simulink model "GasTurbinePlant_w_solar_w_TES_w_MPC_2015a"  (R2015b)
settings: Solver=ode45  StartTime=0.0  StopTime=120  FixedStep=0.05  MinStep=0.000001  RelTol=1e-3
InitFcn:
  | main()
StopFcn:
  | Plot_Step_Test()
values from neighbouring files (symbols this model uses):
  A0 = .945    (= 0.945)    [main.m]
  A1 = -7.8    [main.m]
  A2 = 39    [main.m]
  A_air = (1 - pct) * A_tank    (= 5.890486125)    [main.m]
  A_lm = (A_outer - A_inner) / log(A_outer / A_inner)    [main.m]
  Ac = pct * A_tank    (= 13.744467625)    [main.m]
  B = [-0.22824; 3.3801e5; -3.4738e7; 110.88; -2378.1]    [main.m]
  C = [2.8958e04; 9.3900e03; 3.0120e03; 7.5800e03; 1.4840e03]    [main.m]
  Cp_air = ones(n_tes,1)*300    [main.m]
  Cp_stone = ones(n_tes,1)*1584    [main.m]
  Cpc = 1.005    [main.m]
  Cph = 1.157    [main.m]
  d_rec = 5    [main.m]
  dHst = Hsh - Hcond    (= 811.3)    [main.m]
  dHtot = (Hsh-Hsv)+Hfg+Cpw*delTbfw    (= 2789.54)    [main.m]
  dp = 0.15    [main.m]
  emiss_rec = 0.1    [main.m]
  epsilon = 0.96    [main.m]
  eta_c = 0.86    [main.m]
  eta_comb = 0.99    [main.m]
  eta_HRSG = 0.95    [main.m]
  eta_st = 0.95    [main.m]
  eta_t = 0.89    [main.m]
  F = [1.4250E-06; 5.0390E-01; 1.0830E+02; 0]    [main.m]
  gamma_c = 1.4    [main.m]
  gamma_h = 1.33    [main.m]
  h = ones(n_tes,1)    [main.m]    (also in apm_linprog.m = [hi,hj,hv]'; apm_quadprog.m = [hi,hj,hv]')
  h_node_rec = 2    [main.m]
  k_air = ones(n_tes,1)    [main.m]
  k_stone = 1.7    [main.m]
  LHV = 46000    [main.m]
  m_air = zeros(n_tes,1)    [main.m]
  m_stone = ones(n_tes,1) * V_tank * rho_stone * pct / n_tes    [main.m]
  mu_air2 = zeros(n_tes,1)    [main.m]
  MW_air = 28.97    [main.m]
  n_rec = 10    [main.m]
  n_tes = 10    [main.m]
  Nu = ones(n_tes,1)    [main.m]
  Pa = 101.325    [main.m]
  Pa0 = 101.325    [main.m]
  pct = 0.7    [main.m]
  PR = 15.4    [main.m]
  Pr = ones(n_tes,1)    [main.m]
  q_cond = zeros(n_tes,1)    [main.m]
  q_conv = zeros(n_tes,1)    [main.m]
  q_external = zeros(n_tes,1)    [main.m]
  q_rad = zeros(n_tes,1)    [main.m]
  R = 8.314    [main.m]
  R2 = 0.08206    [main.m]
  Re = ones(n_tes,1)    [main.m]
  rho_air = zeros(n_tes,1)    [main.m]
  SA = 137.445    [main.m]
  sig = 5.6704e-11    [main.m]
  sigma = 5.67e-8    (= 5.67e-08)    [main.m]
  T_air0 = ones(n_tes,1)*298    [main.m]
  T_ref = 298    [main.m]
  T_stone0 = ones(n_tes,1)*298    [main.m]
  T_wall_outer = ones(n_tes,1)*298    [main.m]
  Ta0 = 298.15    [main.m]
  Tao = 298    [main.m]
  theta0 = 11.6    [main.m]
  thetaMAX = 85    [main.m]
  Trec0 = ones(n_rec,1)*550    [main.m]
  U = .010    (= 0.01)    [main.m]
  U_wall = 0.1    [main.m]
  v_air = ones(n_tes,1)    [main.m]
  V_tank = A_tank * len    (= 196.3495375)    [main.m]
  Vol_air = ones(n_tes,1)    [main.m]
  w_rec = 10    [main.m]
  Wfn = 10.2    [main.m]
  Wn = 537    [main.m]
  x = len / n_tes    (= 1)    [main.m]
libraries: simulink x3

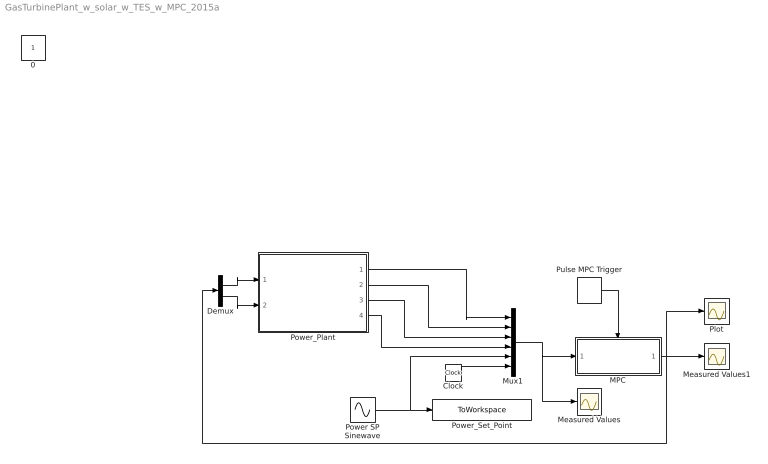
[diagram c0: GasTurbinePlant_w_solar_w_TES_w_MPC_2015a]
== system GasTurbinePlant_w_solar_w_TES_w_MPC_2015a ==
  Clock : Clock
  Demux : Demux  Outputs=2
  MPC : Subsystem  TreatAsAtomicUnit=on
  Measured Values : Scope
  Measured Values1 : Scope
  Mux1 : Mux  Inputs=6
  Plot : Scope
  Power SP Sinewave : Sin  Amplitude=10  Bias=90  Frequency=1/250*20  SampleTime=0
  Power_Plant : Subsystem
  Power_Set_Point : ToWorkspace  VariableName=Power_Set_Point  SaveFormat=Timeseries  SampleTime=-1
  Pulse MPC Trigger : DiscretePulseGenerator  PulseType=Time based  Period=5  PulseWidth=25
  0 : Constant  IOType=siggen
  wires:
  Mux1/1 -> Measured Values/1, MPC/1(In1)
  Pulse MPC Trigger/1 -> MPC/Trigger
  MPC/1(Out1) -> Measured Values1/1, Plot/1, Demux/1
  Demux/1 -> Power_Plant/1(IGV_Input)
  Demux/2 -> Power_Plant/2(Fuel_Input)
  Power_Plant/1(Power_Total) -> Mux1/1
  Power_Plant/3("Te ") -> Mux1/3
  Power_Plant/4("W ") -> Mux1/4
  Clock/1 -> Mux1/6
  Power SP Sinewave/1 -> Power_Set_Point/1, Mux1/5
  Power_Plant/2("Tf ") -> Mux1/2

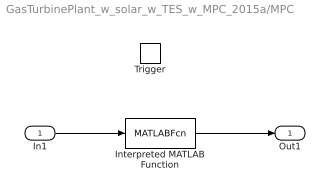
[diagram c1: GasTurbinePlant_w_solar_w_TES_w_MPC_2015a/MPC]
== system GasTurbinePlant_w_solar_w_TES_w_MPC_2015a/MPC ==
  In1 : Inport
  Trigger : TriggerPort
  Interpreted MATLAB Function : MATLABFcn  MATLABFcn=mpc  OutputDimensions=2
  Out1 : Outport  InitialOutput=[50 5]
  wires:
  In1/1 -> Interpreted MATLAB Function/1
  Interpreted MATLAB Function/1 -> Out1/1

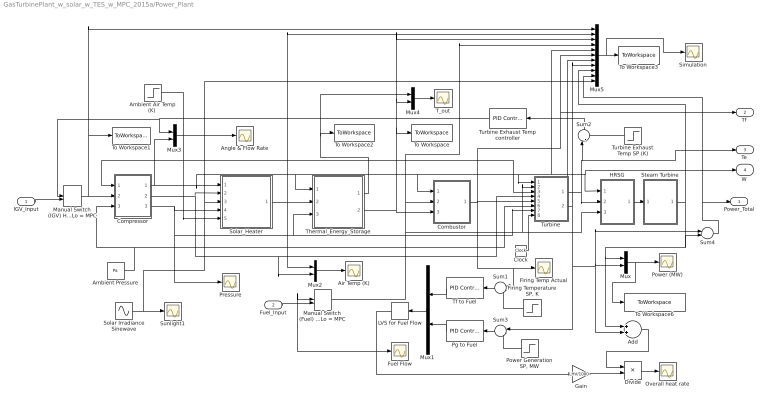
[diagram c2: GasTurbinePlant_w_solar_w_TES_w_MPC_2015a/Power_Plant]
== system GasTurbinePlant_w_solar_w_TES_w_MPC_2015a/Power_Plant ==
  IGV_Input : Inport
  Fuel_Input : Inport  Port=2
  Add : Sum
  Air Temp (K) : Scope
  "Ambient Air Temp (K) " : Step  Time=0  Before=298  After=298  SampleTime=0
  Ambient Pressure : Constant  Value=Pa
  Angle & Flow Rate : Scope
  Clock : Clock
  Combustor : Subsystem
  Compressor : Subsystem
  Divide : Product  Inputs=*/
  Firing Temp Actual : Scope
  "Firing Temperature SP, K" : Step  Time=10  Before=1370  After=1370  SampleTime=0
  Fuel Flow : Scope
  Gain : Gain  Gain=LHV/1000
  HRSG : Subsystem
  LVS for Fuel Flow : MinMax
  Manual Switch (Fuel) Hi = PID Lo = MPC : ManualSwitch  CurrentSetting=0
  Manual Switch (IGV) Hi = PID Lo = MPC : ManualSwitch  CurrentSetting=0
  Mux{,1..4} (5 alike) : Mux  Inputs=2
  Mux5 : Mux  Inputs=11
  Overall heat rate : Scope
  Pg to Fuel : simulink/Continuous/PID Controller  Controller=PID  TimeDomain=Discrete-time  SampleTime=1/60*6  IntegratorMethod=Forward Euler  FilterMethod=Forward Euler  Form=Ideal  UseFilter=on  ControllerParametersSource=internal  P=1/15  I=1  D=0  N=1  InitialConditionSource=internal  InitialConditionForIntegrator=50  InitialConditionForFilter=0  ExternalReset=none  LimitOutput=on  UpperSaturationLimit=12  LowerSaturationLimit=0.5  LinearizeAsGain=off  AntiWindupMode=clamping  Kb=1  TrackingMode=off  Kt=1  PParamMin=[]  PParamMax=[]  IParamMin=[]  IParamMax=[]  DParamMin=[]  DParamMax=[]  NParamMin=[]  NParamMax=[]  KbParamMin=[]  KbParamMax=[]  KtParamMin=[]  KtParamMax=[]  POutMin=[]  POutMax=[]  IOutMin=[]  IOutMax=[]  DOutMin=[]  DOutMax=[]  NOutMin=[]  NOutMax=[]  KbOutMin=[]  KbOutMax=[]  KtOutMin=[]  KtOutMax=[]  IntegratorOutMin=[]  IntegratorOutMax=[]  FilterOutMin=[]  FilterOutMax=[]  SumOutMin=[]  SumOutMax=[]  SumI1OutMin=[]  SumI1OutMax=[]  SumI2OutMin=[]  SumI2OutMax=[]  SumI3OutMin=[]  SumI3OutMax=[]  SumDOutMin=[]  SumDOutMax=[]  SaturationOutMin=[]  SaturationOutMax=[]  IntegratorContinuousStateAttributes=''  IntegratorStateMustResolveToSignalObject=off  IntegratorRTWStateStorageClass=Auto  FilterContinuousStateAttributes=''  FilterStateMustResolveToSignalObject=off  FilterRTWStateStorageClass=Auto  DifferentiatorICPrevScaledInput=0  DifferentiatorOutMin=[]  DifferentiatorOutMax=[]
  Power (MW) : Scope
  "Power Generation SP, MW" : Step  Time=40  Before=230  After=230  SampleTime=0
  Pressure : Scope
  Simulation : Scope
  Solar Irradiance Sinewave : Sin  Amplitude=500  Bias=500  Frequency=1/250*20  SampleTime=0
  Solar_Heater : Subsystem
  Steam Turbine : Subsystem
  Sum1 : Sum  Inputs=|-+
  Sum2 : Sum  Inputs=|-+
  Sum3 : Sum  Inputs=|-+
  Sum4 : Sum  Inputs=|++
  Sunlight1 : Scope
  T_out : Scope
  Tf to Fuel : simulink/Continuous/PID Controller  Controller=PID  TimeDomain=Discrete-time  SampleTime=1/60*6  IntegratorMethod=Forward Euler  FilterMethod=Forward Euler  Form=Ideal  UseFilter=on  ControllerParametersSource=internal  P=1/20  I=1  D=0  N=1  InitialConditionSource=internal  InitialConditionForIntegrator=200  InitialConditionForFilter=0  ExternalReset=none  LimitOutput=on  UpperSaturationLimit=12  LowerSaturationLimit=0.5  LinearizeAsGain=off  AntiWindupMode=clamping  Kb=1  TrackingMode=off  Kt=1  PParamMin=[]  PParamMax=[]  IParamMin=[]  IParamMax=[]  DParamMin=[]  DParamMax=[]  NParamMin=[]  NParamMax=[]  KbParamMin=[]  KbParamMax=[]  KtParamMin=[]  KtParamMax=[]  POutMin=[]  POutMax=[]  IOutMin=[]  IOutMax=[]  DOutMin=[]  DOutMax=[]  NOutMin=[]  NOutMax=[]  KbOutMin=[]  KbOutMax=[]  KtOutMin=[]  KtOutMax=[]  IntegratorOutMin=[]  IntegratorOutMax=[]  FilterOutMin=[]  FilterOutMax=[]  SumOutMin=[]  SumOutMax=[]  SumI1OutMin=[]  SumI1OutMax=[]  SumI2OutMin=[]  SumI2OutMax=[]  SumI3OutMin=[]  SumI3OutMax=[]  SumDOutMin=[]  SumDOutMax=[]  SaturationOutMin=[]  SaturationOutMax=[]  IntegratorContinuousStateAttributes=''  IntegratorStateMustResolveToSignalObject=off  IntegratorRTWStateStorageClass=Auto  FilterContinuousStateAttributes=''  FilterStateMustResolveToSignalObject=off  FilterRTWStateStorageClass=Auto  DifferentiatorICPrevScaledInput=0  DifferentiatorOutMin=[]  DifferentiatorOutMax=[]
  Thermal_Energy_Storage : Subsystem
  To Workspace : ToWorkspace  VariableName=T_stone_out  SaveFormat=Timeseries  SampleTime=-1
  To Workspace1 : ToWorkspace  VariableName=IGV_Angle  SaveFormat=Timeseries  SampleTime=-1
  To Workspace2 : ToWorkspace  VariableName=T_air_out  SaveFormat=Timeseries  SampleTime=-1
  To Workspace3 : ToWorkspace  VariableName=Plant_Data  SaveFormat=Timeseries  SampleTime=-1
  To Workspace6 : ToWorkspace  VariableName=Power  SaveFormat=Timeseries  SampleTime=-1
  Turbine : Subsystem
  Turbine Exhaust Temp SP (K) : Step  Time=40  Before=750  After=750  SampleTime=0
  Turbine Exhaust Temp controller : simulink/Continuous/PID Controller  Controller=PID  TimeDomain=Discrete-time  SampleTime=1/60*6  IntegratorMethod=Forward Euler  FilterMethod=Forward Euler  Form=Parallel  UseFilter=on  ControllerParametersSource=internal  P=-1.5  I=-1  D=0  N=1  InitialConditionSource=internal  InitialConditionForIntegrator=75  InitialConditionForFilter=0  ExternalReset=none  LimitOutput=on  UpperSaturationLimit=88  LowerSaturationLimit=57  LinearizeAsGain=off  AntiWindupMode=clamping  Kb=1  TrackingMode=off  Kt=1  PParamMin=[]  PParamMax=[]  IParamMin=[]  IParamMax=[]  DParamMin=[]  DParamMax=[]  NParamMin=[]  NParamMax=[]  KbParamMin=[]  KbParamMax=[]  KtParamMin=[]  KtParamMax=[]  POutMin=[]  POutMax=[]  IOutMin=[]  IOutMax=[]  DOutMin=[]  DOutMax=[]  NOutMin=[]  NOutMax=[]  KbOutMin=[]  KbOutMax=[]  KtOutMin=[]  KtOutMax=[]  IntegratorOutMin=[]  IntegratorOutMax=[]  FilterOutMin=[]  FilterOutMax=[]  SumOutMin=[]  SumOutMax=[]  SumI1OutMin=[]  SumI1OutMax=[]  SumI2OutMin=[]  SumI2OutMax=[]  SumI3OutMin=[]  SumI3OutMax=[]  SumDOutMin=[]  SumDOutMax=[]  SaturationOutMin=[]  SaturationOutMax=[]  IntegratorContinuousStateAttributes=''  IntegratorStateMustResolveToSignalObject=off  IntegratorRTWStateStorageClass=Auto  FilterContinuousStateAttributes=''  FilterStateMustResolveToSignalObject=off  FilterRTWStateStorageClass=Auto  DifferentiatorICPrevScaledInput=0  DifferentiatorOutMin=[]  DifferentiatorOutMax=[]
  Power_Total : Outport
  "Tf " : Outport  Port=2
  "Te " : Outport  Port=3
  "W " : Outport  Port=4
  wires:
  HRSG/1(msteam) -> Steam Turbine/1(msteam)
  Ambient Pressure/1 -> Turbine/6(Pa), Compressor/3(Pa)
  Combustor/1(Tf) -> Sum1/1, Firing Temp Actual/1, Turbine/5(Tf), Mux5/6, "Tf "/1
  Turbine/1(Te) -> HRSG/2(Te), "Te "/1, Sum2/1, Mux5/7
  "Ambient Air Temp (K) "/1 -> Compressor/1(Ta), Turbine/3(Ti), Solar_Heater/5(Ta)
  Turbine Exhaust Temp controller/1 -> Manual Switch (IGV) Hi = PID Lo = MPC/1, Mux3/1
  Steam Turbine/1(Pst) -> Mux5/9, Sum4/2, Mux/1, Add/1
  Mux/1 -> To Workspace6/1, Power (MW)/1
  Sum2/1 -> Turbine Exhaust Temp controller/1
  Turbine Exhaust Temp SP (K)/1 -> Sum2/2
  Sum1/1 -> Tf to Fuel/1
  "Firing Temperature SP, K"/1 -> Sum1/2
  Turbine/2(Pg) -> Sum3/1, Sum4/1, Mux/2, Add/2, Mux5/8
  Sum3/1 -> Pg to Fuel/1
  "Power Generation SP, MW"/1 -> Sum3/2
  Mux1/1 -> LVS for Fuel Flow/1
  Tf to Fuel/1 -> Mux1/1
  Pg to Fuel/1 -> Mux1/2
  LVS for Fuel Flow/1 -> Manual Switch (Fuel) Hi = PID Lo = MPC/1, Gain/1, Fuel Flow/1
  Add/1 -> Divide/1
  Gain/1 -> Divide/2
  Divide/1 -> Overall heat rate/1
  Compressor/2(Td) -> Mux2/2, Turbine/4(Td), Solar_Heater/2(Td)
  Compressor/1(W) -> Mux3/2, Solar_Heater/1(W), HRSG/1(W), "W "/1, Mux5/5, Turbine/1(W), Combustor/1(W), Thermal_Energy_Storage/1(W)
  Compressor/3(Pd) -> Solar_Heater/4(P), Turbine/7(Pd), Thermal_Energy_Storage/3(P), Pressure/1
  Solar_Heater/1(Tair_out) -> Mux5/2, Mux2/1, Thermal_Energy_Storage/2(T_air_in)
  Mux2/1 -> Air Temp (K)/1
  Thermal_Energy_Storage/2(T_air_out) -> Mux4/2, Mux5/3, To Workspace/1, Combustor/3(Td)
  Thermal_Energy_Storage/1(T_stone_out) -> To Workspace2/1, Mux4/1
  Mux3/1 -> Angle & Flow Rate/1
  Mux4/1 -> T_out/1
  Solar Irradiance Sinewave/1 -> Mux5/11, Solar_Heater/3(q_conc), Sunlight1/1
  Mux5/1 -> To Workspace3/1, Simulation/1
  Manual Switch (IGV) Hi = PID Lo = MPC/1 -> Mux5/1, To Workspace1/1, Compressor/2(thetaIGV)
  Manual Switch (Fuel) Hi = PID Lo = MPC/1 -> HRSG/3(Wf), Turbine/2(Wf), Mux5/4, Combustor/2(Wf)
  IGV_Input/1 -> Manual Switch (IGV) Hi = PID Lo = MPC/2
  Fuel_Input/1 -> Manual Switch (Fuel) Hi = PID Lo = MPC/2
  Sum4/1 -> Mux5/10, Power_Total/1
  Clock/1 -> Turbine/8("clock ")

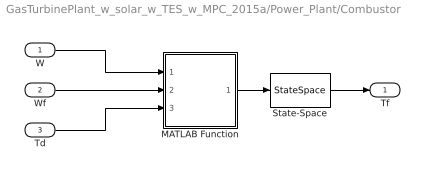
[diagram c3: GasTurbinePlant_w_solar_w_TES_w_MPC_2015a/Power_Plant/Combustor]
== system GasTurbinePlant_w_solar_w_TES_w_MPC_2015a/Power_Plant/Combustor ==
  W : Inport
  Wf : Inport  Port=2
  Td : Inport  Port=3
  MATLAB Function : MATLAB Function  TreatAsAtomicUnit=on
  State-Space : StateSpace  A=-1  D=0  X0=1000
  Tf : Outport
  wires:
  Td/1 -> MATLAB Function/3(Td)
  W/1 -> MATLAB Function/1(W)
  MATLAB Function/1(Tf) -> State-Space/1
  Wf/1 -> MATLAB Function/2(Wf)
  State-Space/1 -> Tf/1

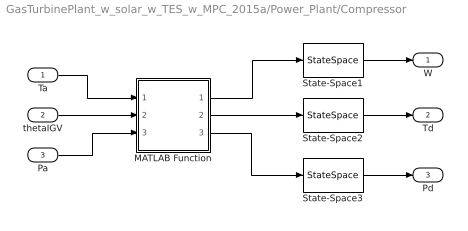
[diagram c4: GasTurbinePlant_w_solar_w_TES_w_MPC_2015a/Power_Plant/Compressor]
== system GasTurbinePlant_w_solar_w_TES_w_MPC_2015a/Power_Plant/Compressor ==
  Ta : Inport
  thetaIGV : Inport  Port=2
  Pa : Inport  Port=3
  MATLAB Function : MATLAB Function  TreatAsAtomicUnit=on
  State-Space1 : StateSpace  A=-1/2  C=1/2  D=0  X0=465
  State-Space2 : StateSpace  A=-1/2  C=1/2  D=0  X0=720
  State-Space3 : StateSpace  A=-1/2  C=1/2  D=0  X0=101.325*PR*2
  W : Outport
  Td : Outport  Port=2
  Pd : Outport  Port=3
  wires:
  MATLAB Function/1(W) -> State-Space1/1
  Pa/1 -> MATLAB Function/3(Pa)
  MATLAB Function/2(Td) -> State-Space2/1
  MATLAB Function/3(Pd) -> State-Space3/1
  thetaIGV/1 -> MATLAB Function/2(thetaIGV)
  Ta/1 -> MATLAB Function/1(Ta)
  State-Space1/1 -> W/1
  State-Space2/1 -> Td/1
  State-Space3/1 -> Pd/1

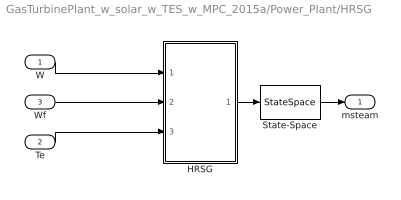
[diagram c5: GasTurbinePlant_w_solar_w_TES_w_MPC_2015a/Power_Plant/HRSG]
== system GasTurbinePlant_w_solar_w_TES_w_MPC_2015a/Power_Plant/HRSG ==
  W : Inport
  Te : Inport  Port=2
  Wf : Inport  Port=3
  HRSG : MATLAB Function  TreatAsAtomicUnit=on
  State-Space : StateSpace  A=-1/4  C=1/4  D=0  X0=44.0853*4
  msteam : Outport
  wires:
  W/1 -> HRSG/1(W)
  HRSG/1(Ms) -> State-Space/1
  State-Space/1 -> msteam/1
  Te/1 -> HRSG/3(Te)
  Wf/1 -> HRSG/2(Wf)

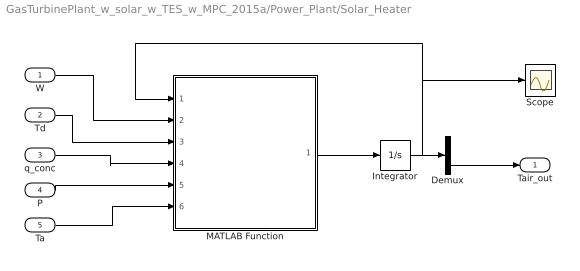
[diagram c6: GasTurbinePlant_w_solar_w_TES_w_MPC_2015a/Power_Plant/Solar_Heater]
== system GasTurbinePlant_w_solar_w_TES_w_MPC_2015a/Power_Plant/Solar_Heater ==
  W : Inport
  Td : Inport  Port=2
  q_conc : Inport  Port=3
  P : Inport  Port=4
  Ta : Inport  Port=5
  Demux : Demux  Outputs=[n_rec-1 1]
  Integrator : Integrator  InitialCondition=Trec0
  MATLAB Function : MATLAB Function  TreatAsAtomicUnit=on
  Scope : Scope
  Tair_out : Outport
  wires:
  MATLAB Function/1(dTdt) -> Integrator/1
  q_conc/1 -> MATLAB Function/4(q_conc)
  P/1 -> MATLAB Function/5(P)
  Ta/1 -> MATLAB Function/6(Ta)
  Integrator/1 -> Scope/1, MATLAB Function/1(T), Demux/1
  Demux/2 -> Tair_out/1
  W/1 -> MATLAB Function/2(W)
  Td/1 -> MATLAB Function/3(Td)

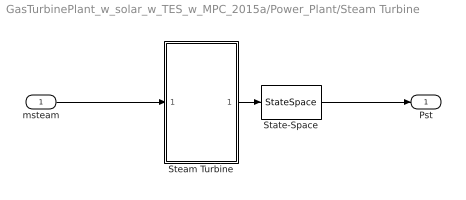
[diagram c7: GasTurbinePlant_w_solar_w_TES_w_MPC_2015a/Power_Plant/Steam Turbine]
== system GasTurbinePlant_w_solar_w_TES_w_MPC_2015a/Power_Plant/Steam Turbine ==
  msteam : Inport
  State-Space : StateSpace  A=-1  D=0  X0=0
  Steam Turbine : MATLAB Function  TreatAsAtomicUnit=on
  Pst : Outport
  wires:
  msteam/1 -> Steam Turbine/1(msteam)
  Steam Turbine/1(Pst) -> State-Space/1
  State-Space/1 -> Pst/1

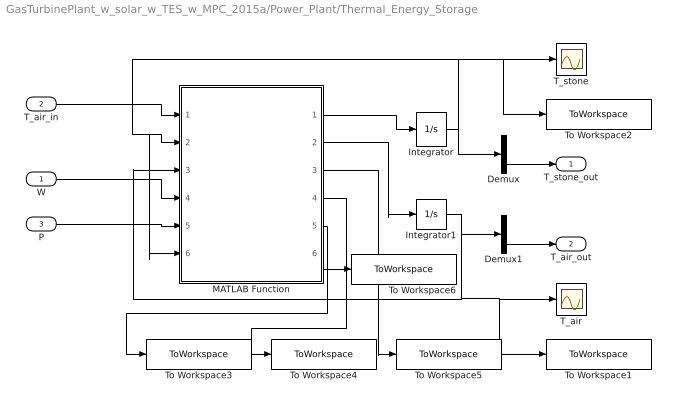
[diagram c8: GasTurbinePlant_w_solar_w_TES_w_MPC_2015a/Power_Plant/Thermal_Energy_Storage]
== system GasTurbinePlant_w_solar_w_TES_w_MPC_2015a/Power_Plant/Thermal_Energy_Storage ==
  W : Inport
  T_air_in : Inport  Port=2
  P : Inport  Port=3
  Demux : Demux  Outputs=[n_tes-1 1]
  Demux1 : Demux  Outputs=[n_tes-1 1]
  Integrator : Integrator  InitialCondition=T_stone0
  Integrator1 : Integrator  InitialCondition=T_air0
  MATLAB Function : MATLAB Function  TreatAsAtomicUnit=on
  T_air : Scope
  T_stone : Scope
  To Workspace1 : ToWorkspace  VariableName=T_air  SaveFormat=Timeseries  SampleTime=-1
  To Workspace2 : ToWorkspace  VariableName=T_stone  SaveFormat=Timeseries  SampleTime=-1
  To Workspace3 : ToWorkspace  VariableName=Radiation  SaveFormat=Timeseries  SampleTime=-1
  To Workspace4 : ToWorkspace  VariableName=Conduction  SaveFormat=Timeseries  SampleTime=-1
  To Workspace5 : ToWorkspace  VariableName=Convection  SaveFormat=Timeseries  SampleTime=-1
  To Workspace6 : ToWorkspace  VariableName=External  SaveFormat=Timeseries  SampleTime=-1
  T_stone_out : Outport
  T_air_out : Outport  Port=2
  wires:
  MATLAB Function/1(dT_stone_dt) -> Integrator/1
  P/1 -> MATLAB Function/5(P)
  Integrator/1 -> MATLAB Function/6(T_wall_inner), MATLAB Function/2(T_stone), To Workspace2/1, T_stone/1, Demux/1
  Demux/2 -> T_stone_out/1
  MATLAB Function/2(dT_air_dt) -> Integrator1/1
  Integrator1/1 -> Demux1/1, To Workspace1/1, T_air/1, MATLAB Function/3(T_air)
  Demux1/2 -> T_air_out/1
  MATLAB Function/3(Convection) -> To Workspace5/1
  MATLAB Function/4(Conduction) -> To Workspace4/1
  MATLAB Function/5(Radiation) -> To Workspace3/1
  W/1 -> MATLAB Function/4(W)
  T_air_in/1 -> MATLAB Function/1(T_air_in)
  MATLAB Function/6(External) -> To Workspace6/1

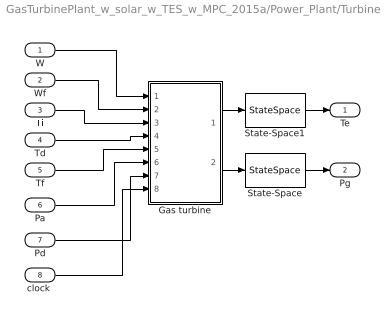
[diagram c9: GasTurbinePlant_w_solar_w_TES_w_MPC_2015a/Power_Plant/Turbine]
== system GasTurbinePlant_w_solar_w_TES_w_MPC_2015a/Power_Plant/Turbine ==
  W : Inport
  Wf : Inport  Port=2
  Ti : Inport  Port=3
  Td : Inport  Port=4
  Tf : Inport  Port=5
  Pa : Inport  Port=6
  Pd : Inport  Port=7
  "clock " : Inport  Port=8
  Gas turbine : MATLAB Function  TreatAsAtomicUnit=on
  State-Space : StateSpace  A=-1  D=0  X0=0
  State-Space1 : StateSpace  A=-1  D=0  X0=298
  Te : Outport
  Pg : Outport  Port=2
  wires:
  W/1 -> Gas turbine/1(W)
  Wf/1 -> Gas turbine/2(Wf)
  Ti/1 -> Gas turbine/3(Ti)
  Td/1 -> Gas turbine/4(Td)
  Tf/1 -> Gas turbine/5(Tf)
  Pa/1 -> Gas turbine/6(Pa)
  Pd/1 -> Gas turbine/7(Pd)
  Gas turbine/1(Te) -> State-Space1/1
  Gas turbine/2(Pg) -> State-Space/1
  State-Space/1 -> Pg/1
  State-Space1/1 -> Te/1
  "clock "/1 -> Gas turbine/8(clock)

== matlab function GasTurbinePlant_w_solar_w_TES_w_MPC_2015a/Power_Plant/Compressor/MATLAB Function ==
function [W, Td, Pd] = compressor(Ta, thetaIGV, Pa, Ta0, Pa0, theta0,...
    A0, A1, A2, thetaMAX, gamma_c, Wn, eta_c, PR)

%global Ta0 Pa0 theta0 A0 A1 A2 thetaMAX

N=1;

DNc = abs(N*sqrt(Ta0/Ta)-1); % Added abs() to avoid negative (and imaginary) numbers

UDNc = 1+A0*DNc+A1*DNc^2+A2*DNc^3;

W = (UDNc*Pa/Pa0*sqrt(Ta0/Ta)*...
    sind(thetaIGV-theta0)/sind(thetaMAX-theta0)*Wn);

xc = (PR*W/Wn)^((gamma_c-1)/gamma_c); %Intermediate variable

Td = Ta*(1+(xc-1)/eta_c); %Compressor discharge temp

Pd = Pa*PR; %compressor discharge pressure

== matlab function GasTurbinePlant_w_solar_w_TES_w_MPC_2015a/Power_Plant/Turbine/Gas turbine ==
function [Te, Pg] = turbine(W, Wf, Ti, Td, Tf, Pa, Pd, Wn, Cph, Wfn,...
    gamma_h, eta_t, Cpc, clock)


PR = Pd/Pa;

xh = (PR*(Wfn+W)/(Wfn+Wn))^((gamma_h-1)/gamma_h);

Te = Tf*(1-(1-1/xh)*eta_t); %Exhaust temp

Pg = (W+Wf)*Cph*(Tf-Te) - W*Cpc*(Td-Ti); %Power generation, kW
Pg = Pg/1000; %MW

% Code for breakpoint
if clock >= 4
    PR = PR;
end

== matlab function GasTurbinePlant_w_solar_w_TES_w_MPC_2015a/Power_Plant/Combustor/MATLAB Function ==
function Tf  = combustor(W, Wf, Td, Cph, LHV, eta_comb)

Tf = Td + (eta_comb*LHV/Cph)*(Wf/(Wf+W)); %Firing temp (K)

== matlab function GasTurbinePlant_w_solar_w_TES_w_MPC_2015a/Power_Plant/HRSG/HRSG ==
function Ms = HRSG(W, Wf, Te, Cpc, eta_HRSG, dHtot, Tao)

Ms = (eta_HRSG*Cpc*(W+Wf)*(Te-Tao))/dHtot;

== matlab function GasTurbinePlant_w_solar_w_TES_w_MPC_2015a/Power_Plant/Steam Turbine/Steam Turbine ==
function Pst = steamturbine(msteam, eta_st, dHst)

Pst = eta_st*msteam*dHst; %steam turbine power output, kW

Pst = Pst/1000; %steam turbine power output, MW

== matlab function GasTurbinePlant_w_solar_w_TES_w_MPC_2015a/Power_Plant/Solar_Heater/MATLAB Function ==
function dTdt = solar_receiver(T, W, Td, q_conc, P, Ta, sig, emiss_rec,...
    MW_air, h_node_rec, w_rec, d_rec, U, R, Cph)
%#codegen

Vnode = w_rec*h_node_rec*d_rec; %m^3, node volume
rho = P*MW_air./(R*T); %kg/m^3, air density

dTdt = zeros(size(T)); %set initial size of dTdt and populate with zeros

    dTdt(1) = 60/(rho(1)*Vnode*Cph)*(W*Cph*(Td-T(1))+...
        q_conc*h_node_rec*w_rec - ...
        sig*emiss_rec*(T(1)^4-Ta^4)*h_node_rec*w_rec -...
        U*h_node_rec*w_rec*(T(1)-Ta));

    %K/min, energy balance on node 1 (the first node)

for i =2:length(T)
    
    dTdt(i) = 60/(rho(i)*Vnode*Cph)*(W*Cph*(T(i-1)-T(i))+...
        q_conc*h_node_rec*w_rec - ...
        sig*emiss_rec*(T(i)^4-Ta^4)*h_node_rec*w_rec -...
        U*h_node_rec*w_rec*(T(i)-Ta));
    
    %K/min, energy balance on nodes 2-n_rec. Air exits at the temperature of 
    %the last node (n_rec)
    k=1;
end

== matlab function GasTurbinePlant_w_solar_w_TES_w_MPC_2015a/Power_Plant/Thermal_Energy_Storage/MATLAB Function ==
function [dT_stone_dt, dT_air_dt, Convection, Conduction, Radiation, External] = thermal_energy_storage(T_air_in, T_stone, ...
    T_air, W, P, MW_air, Cp_air, Cp_stone, rho_air, m_air, m_stone, q_cond, q_conv, q_rad, Nu, Pr, Re, ...
    R, R2, T_ref, k_stone, k_air, mu_air2, sigma, epsilon, V_tank, pct, Ac, SA, x, n_tes, B, C, E, F, ...
    A_air, dp, h, Vol_air, v_air, T_wall_inner, T_wall_outer, q_external, U_wall, A_lm)

%Cp_air_in = 300; % J/kg-K
Cp_air_in = (C(1)+C(2)*(C(3)/T_air_in/sinh(C(3)/T_air_in))^2+C(4)*(C(5)/T_air_in/cosh(C(5)/T_air_in))^2)/MW_air; % J/kg-K
%	T_air_in = 1373.15				% K (1100 C)
%rho_air_in = MW_air * P / (R2 * T_air_in);	% kg/m^3 (Verify these units…)
%V_air_in = W / rho_air_in; % = 15 * 60 %* 100			% m3/sec —> Converted to per min (but actually still in per sec)

for i = 1:n_tes %length(T_air) % Get clarification about T; also initial value definitions; start at 2 or 1?
    
    Cp_air(i) = (C(1)+C(2)*((C(3)/T_air(i))/sinh(C(3)/T_air(i)))^2+C(4)*((C(5)/T_air(i))/cosh(C(5)/T_air(i)))^2)/MW_air; % J/kg-K = (J/kmol-K)/(kg/kmol)      %Cp_air(i) = 300; % J/kg-K
    rho_air(i) = MW_air * P / (R * T_air(i)); % (kg/m^3)
    m_air(i) = V_tank * (1 - pct) * rho_air(i) / n_tes;	% Mass of air in each slice % Is this correct? Do a mass balance eqn for air.
    Cp_stone(i) = (B(1)+B(2)*T_stone(i)^(-2)+B(3)*T_stone(i)^(-3)+B(4)*T_stone(i)^(-0.5)+B(5)*T_stone(i)^(-1))*1000; % J/kg-K      %Cp_stone(i) = 1584; % J/kg-K  

    Vol_air(i) = W / rho_air(i) / 60; % Volumetric flow rate (m^3/s)
    v_air(i) = Vol_air(i) / A_air; % Velocity of air (m/s)
    mu_air2(i) = F(1)*T_air(i)^F(2) / (1 + F(3)/T_air(i) + F(4)/T_air(i)^2); % Viscosity of air (kg/m/s = Pa*s)    

    % External heat loss
    T_wall_inner(i) = T_stone(i);
    q_external(i) = U_wall * A_lm * (T_wall_inner(i) - T_wall_outer(i));
    
    % Heat transfer coefficient correlation
    k_air(i) = (E(1)*T_air(i)^E(2))/(1+E(3)/T_air(i)+E(4)/T_air(i)^2); % Thermal conductivity of air    
    Pr(i) = ( Cp_air(i) * mu_air2(i) ) / k_air(i); % Cp_air definition already includes 1/MW_air      %Pr(i) = 0.7;
    Re(i) = rho_air(i) * dp * v_air(i) / mu_air2(i);
    Nu(i) = (1/3 * (3/2 * Re(i))^(1/2) + 2/15 * (3/2 * Re(i))^(2/3)) * Pr(i)^(1/3);
    h(i) = Nu(i)*k_air(i)/dp; % Convection coefficient   %h(i) = 30;    
    
    % Old Heat Transfer Coefficient
    %G = air flow rate (lb/hr/m^2)
    %GD = W / A_air / dp * 2.204621 / 3.28084^3 * 3600; % lb/hr-ft3
    %h = 0.652 * GD^0.7 * 0.29307 * 3.28084^3 / 1.8; % W/m3-K
    %h = 12;
    
    %Conduction
    %q_cond(1) = k_stone * Ac / x * (T_stone(1) - T_stone(2));
    if i == length(T_air)
        q_cond(i) = 0;
    else
        q_cond(i) = 60 * (k_stone * Ac / x * (T_stone(i) - T_stone(i+1)));  % 60 converts to per minute
    end
    
    % Convection —> Need to include heat transfer between the hot air and cold air somehow (?)
    q_conv(i) = 60 * (h(i) * SA * (T_air(i) - T_stone(i)));
    
    % Radiation —> There is an issue here, because as the grid size shrinks the effect of radiation is minimized (?)
    q_rad(i) = 60 * (epsilon * sigma * SA * (T_air(i)^4 - T_stone(i)^4));
    
    
end

Convection = q_conv;
Conduction = q_cond;
Radiation = q_rad;
External = q_external;


%Equations
    dT_stone_dt = zeros(size(T_stone));
    dT_stone_dt(1) = (q_conv(1) - q_cond(1) + q_rad(1)) / ...
        (m_stone(1) * Cp_stone(1));
    
    dT_air_dt = zeros(size(T_air));
    dT_air_dt(1) = (W * Cp_air_in * (T_air_in - T_ref) - ...
        W * Cp_air(1) * (T_air(1) - T_ref) - q_conv(1) - ...
        q_rad(1)) / (m_air(1) * Cp_air(1));

for i = 2:length(T_stone)
    dT_stone_dt(i) = (q_conv(i) + q_cond(i-1) - q_cond(i) + q_rad(i)) / ...
        (m_stone(i) * Cp_stone(i));
    if i == length(T_stone)
        dT_stone_dt(i) = (q_conv(i) + q_cond(i-1) + q_rad(i)) / ...
            (m_stone(i) * Cp_stone(i));
    end
    dT_air_dt(i) = (W * Cp_air(i-1) * (T_air(i-1) - T_ref) - ...
        W * Cp_air(i) * (T_air(i) - T_ref) - q_conv(i) - ...
        q_rad(i)) / (m_air(i) * Cp_air(i));
end
